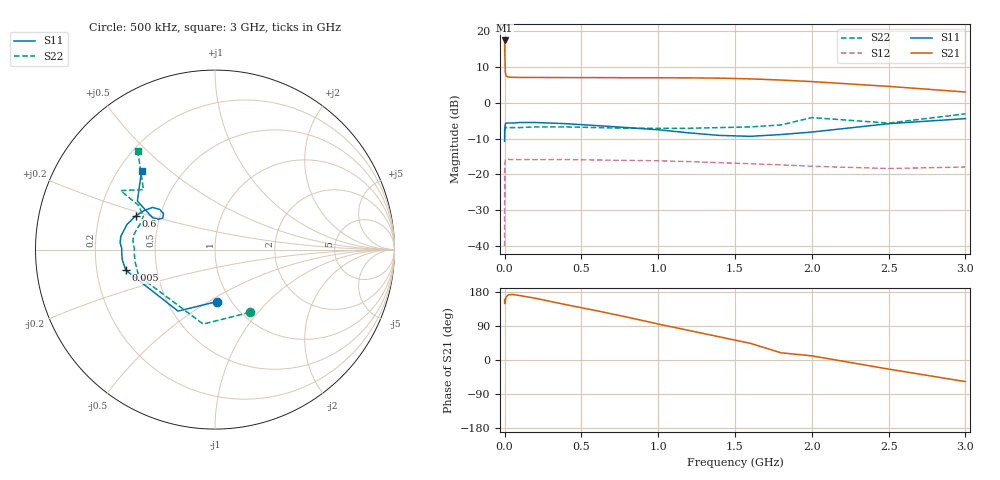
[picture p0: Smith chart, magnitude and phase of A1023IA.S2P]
!  MSA1023 S PARAMETERS
!  Id=325 mA  LAST UPDATED 07-27-92
# ghz s ma r 50
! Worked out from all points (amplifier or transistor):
!   19 points, 500 kHz to 3 GHz, reference 50 ohm
!   highest |S21| = 17.4 dB at 500 kHz (marker M1)
!   |S21| within 3 dB of that: start of sweep to 1.577 MHz
!   unconditionally stable (mu >= 1): start of sweep to 859 kHz; 4.288 MHz to 1.948 GHz; 2.162 GHz to 2.675 GHz
!   at 10 MHz: K = 1.16, MAG = 9.2 dB, |S12| = -15.8 dB
!   at 600 MHz: K = 1.23, MAG = 8.6 dB, |S12| = -16.0 dB
!   at 3 GHz: K = 0.60, MSG = 10.5 dB, |S12| = -17.9 dB
!   S11 on the Smith chart (normalised r, x): 500 kHz: 0.86, -0.54; 5 MHz: 0.33, -0.10; 600 MHz: 0.36, +0.18; 3 GHz: 0.29, +0.40
0.0005  0.29 -88.0  7.38 160.0  0.01 25.0  0.4 -61.0
0.001  0.4 -121.0  5.85 149.0  0.128 22.0  0.42 -99.0
0.005  0.51 -167.0  2.67 156.0  0.16 6.0  0.45 -161.0
0.01  0.52 -174.0  2.36 166.0  0.162 3.0  0.45 -171.0
0.025  0.52 -178.0  2.28 172.0  0.162 1.0  0.45 -177.0
0.05  0.52 179.0  2.26 173.0  0.161 -1.0  0.45 -179.0
0.1  0.53 176.0  2.25 170.0  0.161 -3.0  0.45 179.0
0.2  0.53 172.0  2.25 163.0  0.161 -5.0  0.46 174.0
0.4  0.51 164.0  2.24 146.0  0.161 -11.0  0.46 170.0
0.6  0.48 157.0  2.24 130.0  0.159 -16.0  0.45 165.0
0.8  0.45 151.0  2.23 113.0  0.157 -21.0  0.44 161.0
1  0.42 146.0  2.23 95.0  0.155 -26.0  0.44 157.0
1.2  0.38 144.0  2.22 78.0  0.151 -31.0  0.44 155.0
1.4  0.35 145.0  2.2 61.0  0.146 -36.0  0.45 154.0
1.6  0.34 149.0  2.15 44.0  0.141 -41.0  0.46 153.0
1.8  0.36 152.0  2.07 19.0  0.136 -45.0  0.49 150.0
2  0.39 153.0  1.97 11.0  0.13 -49.0  0.62 148.0
2.5  0.51 148.0  1.69 -24.0  0.121 -52.0  0.52 140.0
3  0.6 133.0  1.41 -57.0  0.127 -57.0  0.7 128.0
